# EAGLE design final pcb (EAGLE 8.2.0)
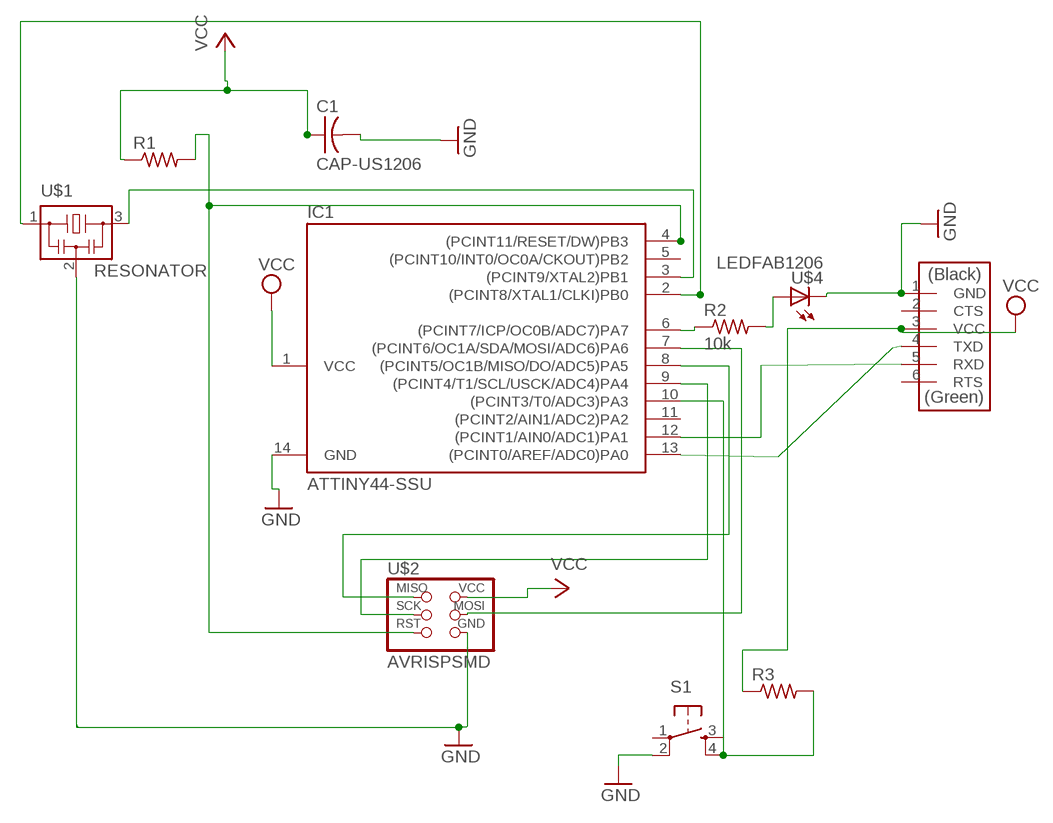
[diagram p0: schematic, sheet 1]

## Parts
C1  CAP-US1206  [C1206]
IC1  ATTINY44-SSU  [SOIC14]
R1  RES-US1206FAB  [R1206FAB]
R2  10k  RES-US1206  [R1206]
R3  RES-US1206  [R1206]
S1  6MM_SWITCH6MM_SWITCH  [6MM_SWITCH]
U$1  RESONATOR  [EFOBM]
U$2  AVRISPSMD  [2X03SMD]
U$3  FTDI-SMD-HEADER  [1X06SMD]
U$4  LEDFAB1206  [LED1206FAB]

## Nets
GND: C1.2 IC1.14(GND) S1.2(P1) U$1.2 U$2.6(GND) U$3.1(GND) U$4.2(C)
N$1: IC1.4((PCINT11/RESET/DW)PB3) R1.2 U$2.5(RST)
N$2: IC1.6((PCINT7/ICP/OC0B/ADC7)PA7) R2.1
N$3: R2.2 U$4.1(A)
N$4: IC1.13((PCINT0/AREF/ADC0)PA0) U$3.4(TXD)
N$5: IC1.12((PCINT1/AIN0/ADC1)PA1) U$3.5(RXD)
N$6: IC1.9((PCINT4/T1/SCL/USCK/ADC4)PA4) U$2.3(SCK)
N$7: IC1.8((PCINT5/OC1B/MISO/DO/ADC5)PA5) U$2.1(MISO)
N$12: IC1.2((PCINT8/XTAL1/CLKI)PB0) U$1.1
N$13: IC1.3((PCINT9/XTAL2)PB1) U$1.3
N$14: IC1.7((PCINT6/OC1A/SDA/MOSI/ADC6)PA6) U$2.4(MOSI)
RESET: IC1.10((PCINT3/T0/ADC3)PA3) R3.2 S1.4(S1)
VCC: C1.1 IC1.1(VCC) R1.1 R3.1 U$2.2(VCC) U$3.3(VCC)
Unconnected: IC1.5((PCINT10/INT0/OC0A/CKOUT)PB2) IC1.11((PCINT2/AIN1/ADC2)PA2) S1.1(P) S1.3(S) U$3.2(CTS) U$3.6(RTS)

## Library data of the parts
C1 = fab:CAP-US
IC1 = fab:ATTINY44
R1-R3 = fab:RES-US: Resistor (US Symbol)
S1 = fab:6MM_SWITCH: OMRON SWITCH
U$1 = fab:RESONATOR
U$2 = fab:AVRISP
U$3 = fab:FTDI-SMD-HEADER
U$4 = fab:LED: LED

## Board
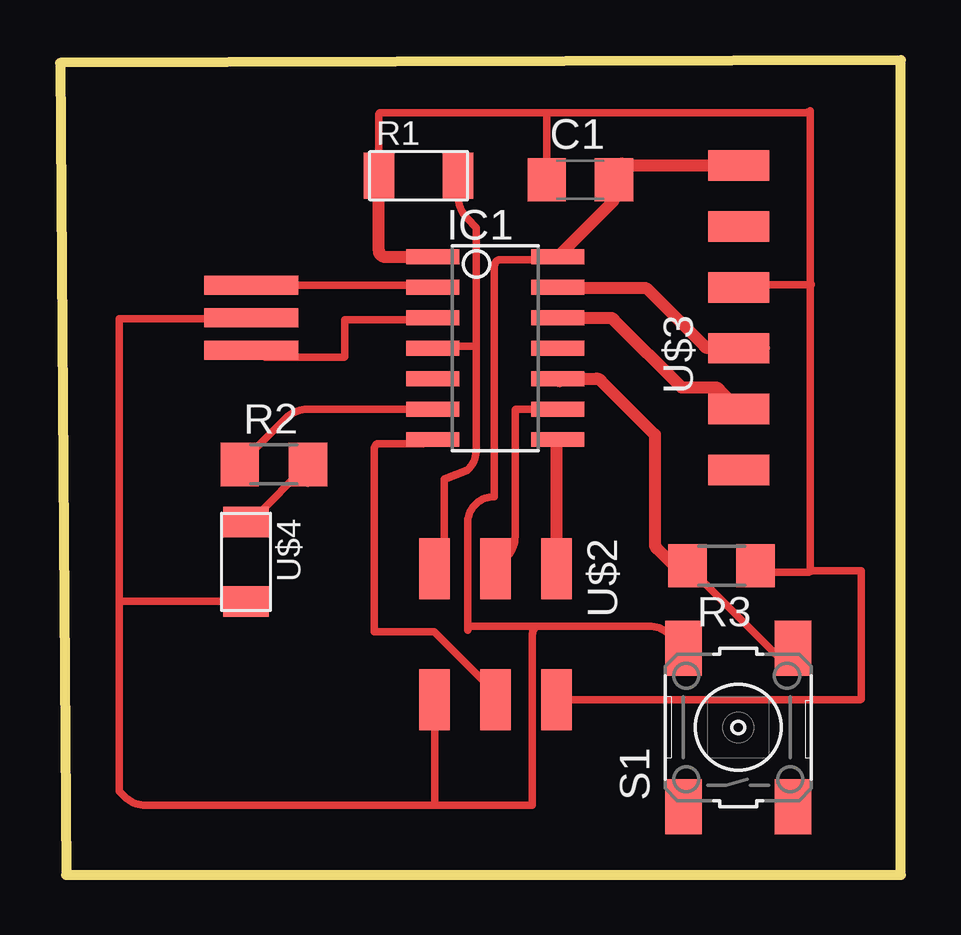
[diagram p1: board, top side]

Size 35.04 x 33.95 mm. Coordinates in mm from the lower left corner, seen from the top.
Outline: 0.25,0 35.04,0 35.04,33.95 0,33.83 0.25,0
Copper layers (1*16): Top 0.035mm / dielectric 1.5mm / Bottom 0.035mm
Design rules "default": minimum track width 10mil, minimum drill 24mil, track to track 8mil, track to pad 8mil, pad to pad 8mil, via to via 8mil, smd to smd 8mil, copper to edge 40mil, drill to drill 8mil, minimum pad ring 10mil, minimum via ring 8mil, stop-mask expansion 4mil, vias tented up to drill 0mil, thermal gap 10mil

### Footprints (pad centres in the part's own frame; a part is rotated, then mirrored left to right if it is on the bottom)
C1206 = smd 1.6 x 1.8: 1 -1.4,0; 2 1.4,0
SOIC14 = smd 0.61 x 2.21: 1 -3.81,-2.603; 2 -2.54,-2.603; 3 -1.27,-2.603; 4 0,-2.603; 5 1.27,-2.603; 6 2.54,-2.603; 7 3.81,-2.603; 8 3.81,2.603; 9 2.54,2.603; 10 1.27,2.603; 11 0,2.603; 12 -1.27,2.603; 13 -2.54,2.603; 14 -3.81,2.603
R1206FAB = smd 1.27 x 1.905: 1 -1.651,0; 2 1.651,0
R1206 = smd 1.6 x 1.803: 1 -1.422,0; 2 1.422,0
6MM_SWITCH = smd 2.286 x 1.524: 1 -3.302,2.286; 2 3.302,2.286; 3 -3.302,-2.286; 4 3.302,-2.286
EFOBM = smd 0.8 x 3.9: 1 -1.35,0; 2 0,0; 3 1.35,0
2X03SMD = smd 2.54 x 1.27: 1 -2.54,2.54; 2 2.92,2.54; 3 -2.54,0; 4 2.92,0; 5 -2.54,-2.54; 6 2.92,-2.54
1X06SMD = smd 2.54 x 1.27: 1 0,6.35; 2 0,3.81; 3 0,1.27; 4 0,-1.27; 5 0,-3.81; 6 0,-6.35
LED1206FAB = smd 1.27 x 1.905: 1 -1.651,0; 2 1.651,0

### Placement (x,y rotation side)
C1  21.68,28.96 0 top
IC1  18.13,21.94 270 top
R1  14.94,29.13 0 top
R2  8.91,17.1 0 top
R3  27.56,12.88 180 top
S1  28.26,6.14 90 top
U$1  7.97,23.21 270 top
U$2  18.15,10.22 270 top
U$3  28.29,23.21 0 top
U$4  7.75,13.04 270 top

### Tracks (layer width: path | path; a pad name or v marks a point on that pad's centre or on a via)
GND
  Top 0.305: IC1.14 arc-90 20.61,25.63 18.35,25.63 arc90 18.1,25.38 18.1,15.76 arc90 16.98,14.64 16.98,10.36 | 16.98,10.36 16.98,10.19 | S1.2 25.43,9.99 arc45 24.53,10.36 19.85,10.36 | 19.85,10.36 16.98,10.36 | U$1.2 arc-45 7.85,23.16 2.46,23.16 2.46,11.46 | 2.46,11.46 2.46,3.49 2.69,3.26 arc45 3.59,2.89 15.69,2.89 | 15.69,2.89 19.67,2.89 19.67,9.92 arc-45 19.85,10.36 | U$4.2 2.63,11.39 arc-45 2.46,11.46 | U$2.6 15.61,3.08 arc45 15.69,2.89
  Top 0.508: 29.04,29.56 23.33,29.56 arc90 23.08,29.31 C1.2 23.08,28.2 arc-45 23.01,28.02 IC1.14
  Top 0.61: 23.41,29.59 arc45 C1.2 | 29.11,29.59 arc-45 29.04,29.56 U$3.1
N$1
  Top 0.254: 14.78,21.91 15.46,21.91 IC1.4
  Top 0.305: R1.2 16.59,28.26 arc45 16.96,27.36 17.35,26.97 17.35,22.03 | 17.35,22.03 17.35,17.75 arc-45 16.98,16.85 16.02,16.49 16.02,13.77 arc-90 U$2.5 | IC1.4 arc-90 15.62,22.03 17.35,22.03
N$2
  Top 0.305: 15.41,19.52 IC1.6 10.31,19.4 arc45 9.42,19.03 R2.1
N$3
  Top 0.305: 10.33,16.32 R2.2 8.05,14.81 arc-45 U$4.1
N$4
  Top 0.508: IC1.13 arc90 20.78,24.43 24.44,24.43 26.86,22.01 arc45 27.03,21.94 U$3.4 29.33,21.94
  Top 0.61: U$3.4 28.18,22.05 28.18,21.64
N$5
  Top 0.508: IC1.12 22.89,23.21 arc-45 23.07,23.14 25.9,20.31 27.28,20.31 arc-45 27.45,20.24 U$3.5
N$6
  Top 0.254: IC1.9 21.41,19.4
  Top 0.305: U$2.3 18.59,13.2 arc45 18.96,14.1 18.96,19.37 arc-45 19.03,19.4 IC1.9
N$7
  Top 0.508: U$2.1 20.69,18.09 arc-90 IC1.8
N$12
  Top 0.305: IC1.2 arc45 15.33,24.56 U$1.1
  Top 0.406: 15.45,24.56 arc-90 IC1.2
  Top 0.508: U$1.1 arc90 8.05,24.48
N$13
  Top 0.305: IC1.3 arc-90 15.45,23.13 11.87,23.13 11.87,21.61 arc-90 11.82,21.56 8.56,21.56 arc90 8.26,21.86 U$1.3
N$14
  Top 0.305: 17.97,7.74 arc-45 U$2.4 | 18.35,8.13 18.35,7.78 arc-45 U$2.4 | U$2.4 arc45 17.96,7.76 15.59,10.13 13.09,10.13 13.09,17.68 arc-45 13.21,17.97 15.14,17.97 arc45 IC1.7
RESET
  Top 0.305: R3.2 29.83,9.19 arc45 30.72,8.82 31.05,8.82 30.63,9.24 arc-45 S1.4
  Top 0.508: 20.83,20.57 arc-90 IC1.10 22.36,20.67 arc-45 22.53,20.6 24.79,18.34 24.79,13.78 arc45 24.86,13.6 26.14,12.33 R3.2
  Top 0.61: 21.73,20.67 IC1.10
VCC
  Top 0.254: 20.26,29.23 C1.1
  Top 0.305: R1.1 13.29,31.66 arc-45 13.33,31.76 20.2,31.76 | 20.2,31.76 31.09,31.76 arc45 31.26,31.83 31.26,24.69 | 31.26,24.69 arc45 31.3,24.59 28.56,24.59 arc45 U$3.3 | C1.1 20.28,31.57 arc45 20.2,31.76 | 31.26,24.69 31.26,12.77 arc-45 31.19,12.6 | 31.19,12.6 29.66,12.6 arc-45 R3.1 | U$2.2 33.32,7.3 arc45 33.39,7.33 33.39,12.66 31.34,12.66 arc45 31.19,12.6
  Top 0.508: R1.1 13.29,26 arc90 13.54,25.75 IC1.1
